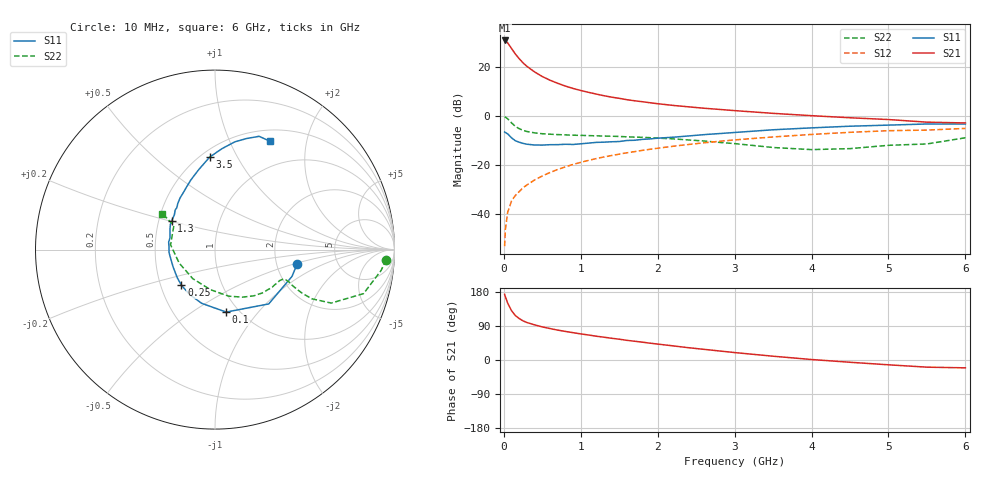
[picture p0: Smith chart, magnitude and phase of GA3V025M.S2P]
! Infineon Technologies  Discrete & RF Semiconductors
! BF775
! Si NPN RF Bipolar Junction Transistor in SOT23
! VCE = 3 V  IC = 25 mA
! Common Emitter S-Parameters:  May  1996
# GHz  S  MA  R  50
!  f  S11  S21  S12  S22
! GHz  MAG  ANG  MAG  ANG  MAG  ANG  MAG  ANG
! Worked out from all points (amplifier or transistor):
!   36 points, 10 MHz to 6 GHz, reference 50 ohm
!   highest |S21| = 30.6 dB at 10 MHz (marker M1)
!   |S21| within 3 dB of that: start of sweep to 93.98 MHz
!   unconditionally stable (mu >= 1): 301.8 MHz to 3.195 GHz
!   at 250 MHz: K = 0.94, MSG = 25.4 dB, |S12| = -29.3 dB
!   at 1.4 GHz: K = 1.14, MAG = 9.7 dB, |S12| = -16.2 dB
!   at 6 GHz: K = 0.98, MSG = 1.1 dB, |S12| = -5.2 dB
!   S11 on the Smith chart (normalised r, x): 10 MHz: 2.61, -0.53; 100 MHz: 0.88, -0.70; 250 MHz: 0.64, -0.27; 1.3 GHz: 0.58, +0.20; 3.5 GHz: 0.55, +0.78; 6 GHz: 0.64, +1.42
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0.01  0.465 -9.8  34.04 173.4  0.0022 83.6  0.9548 -3.4
0.02  0.4543 -19.2  33.42 166.9  0.0048 82.2  0.9324 -7.2
0.05  0.4257 -45.3  30.34 150.1  0.0108 73.7  0.8632 -16.5
0.1  0.3536 -79.8  23.35 130.1  0.0183 67.1  0.7129 -24.7
0.15  0.3086 -103.8  18 117.2  0.0238 65.5  0.6064 -26.9
0.2  0.2878 -119.2  14.45 109.3  0.0285 67.5  0.5438 -26.6
0.25  0.2728 -133.3  11.89 103.3  0.0341 68.0  0.5025 -25.7
0.3  0.2624 -143.1  10.11 98.9  0.0388 69.7  0.4766 -24.9
0.4  0.2526 -157.4  7.778 92.7  0.049 70.6  0.4464 -23.5
0.5  0.2518 -168.2  6.273 87.3  0.0591 71.6  0.4289 -23.1
0.6  0.2565 -176.2  5.276 83.0  0.0696 71.6  0.4195 -23.1
0.7  0.2571 176.0  4.563 78.9  0.0802 71.7  0.4121 -23.7
0.8  0.2616 170.8  4.008 75.4  0.0906 70.8  0.4061 -24.5
0.9  0.2592 165.0  3.585 72.1  0.1017 70.3  0.4007 -25.4
1.1  0.2763 155.2  2.989 66.0  0.1229 68.9  0.3929 -28.3
1.3  0.2886 147.0  2.552 60.2  0.1442 67.1  0.3846 -31.2
1.6  0.3127 135.2  2.116 51.9  0.1753 64.0  0.3709 -36.7
2.2  0.3642 118.8  1.618 37.3  0.2384 57.2  0.3371 -49.7
3.5  0.5163 93.3  1.115 10.0  0.3689 40.3  0.2247 -96.5
4.5  0.6103 79.6  0.907 -6.0  0.4585 26.3  0.2133 -159.4
5.5  0.6775 68.7  0.738 -18.9  0.5086 11.0  0.2657 149.5
6  0.6766 63.2  0.711 -20.7  0.5508 6.6  0.3549 145.6
